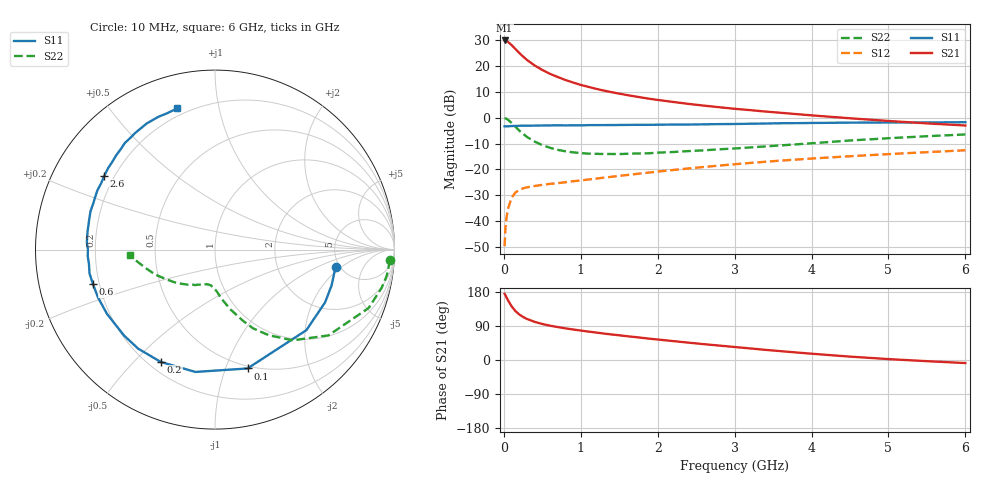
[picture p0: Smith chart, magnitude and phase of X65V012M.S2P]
! SIEMENS Small Signal Semiconductors
! BFP193W
! Si NPN RF Bipolar Junction Transistor in SOT343
! VCE = 5 V  IC = 12 mA
! Common Emitter S-Parameters:  April 1994
# GHz  S  MA  R  50
!  f  S11  S21  S12  S22
! GHz  MAG  ANG  MAG  ANG  MAG  ANG  MAG  ANG
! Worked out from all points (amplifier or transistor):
!   40 points, 10 MHz to 6 GHz, reference 50 ohm
!   highest |S21| = 29.8 dB at 10 MHz (marker M1)
!   |S21| within 3 dB of that: start of sweep to 141.1 MHz
!   unconditionally stable (mu >= 1): 1.244 GHz to 4.268 GHz
!   at 200 MHz: K = 0.25, MSG = 26.5 dB, |S12| = -28.0 dB
!   at 1.5 GHz: K = 1.07, MAG = 14.2 dB, |S12| = -22.5 dB
!   at 6 GHz: K = 0.92, MSG = 4.8 dB, |S12| = -12.6 dB
!   S11 on the Smith chart (normalised r, x): 10 MHz: 4.59, -1.67; 100 MHz: 0.48, -1.19; 200 MHz: 0.25, -0.60; 600 MHz: 0.18, -0.14; 2.6 GHz: 0.16, +0.30; 6 GHz: 0.16, +0.76
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0.01  0.6785 -8.3  30.81 174.7  0.0033 88.0  0.9769 -3.5
0.02  0.6796 -17.2  30.78 171.2  0.0072 80.7  0.9677 -8.7
0.03  0.6801 -25.7  30.38 167.1  0.0102 80.1  0.9532 -12.8
0.05  0.6788 -41.4  29.23 158.9  0.0166 71.6  0.916 -20.8
0.1  0.6866 -74.7  25.2 142.0  0.0282 57.6  0.7923 -37.1
0.15  0.6903 -99.1  21.14 129.2  0.0357 47.9  0.666 -49.4
0.2  0.6951 -115.7  17.69 120.2  0.04 42.0  0.5628 -57.9
0.25  0.6985 -127.8  15.09 113.6  0.0431 38.1  0.4873 -64.2
0.3  0.6971 -136.6  12.99 108.4  0.045 36.2  0.4241 -68.7
0.4  0.7004 -149.2  10.16 100.7  0.0479 33.7  0.3444 -75.5
0.5  0.7044 -157.9  8.302 95.0  0.0503 33.8  0.2943 -80.3
0.6  0.7065 -164.1  6.991 90.6  0.0526 34.0  0.2614 -84.0
0.8  0.7067 -173.5  5.318 83.5  0.0566 36.0  0.224 -89.3
1.1  0.7148 177.0  3.918 75.0  0.0639 39.9  0.2015 -96.0
1.3  0.7173 171.6  3.322 69.8  0.0693 42.1  0.1985 -99.8
1.6  0.7226 164.9  2.726 62.8  0.078 44.5  0.2 -104.9
2.2  0.7337 153.3  2.005 49.9  0.0973 47.2  0.2165 -115.7
2.6  0.7414 146.3  1.703 41.8  0.1114 47.6  0.2332 -123.0
3.2  0.7609 136.3  1.394 30.6  0.1331 46.5  0.2654 -134.0
4.5  0.7992 118.4  0.97 8.9  0.1795 41.0  0.3614 -157.5
5.5  0.8052 109.3  0.773 -3.1  0.2151 35.8  0.4372 -171.1
6  0.8146 104.9  0.704 -8.1  0.2343 33.3  0.4728 -176.5
